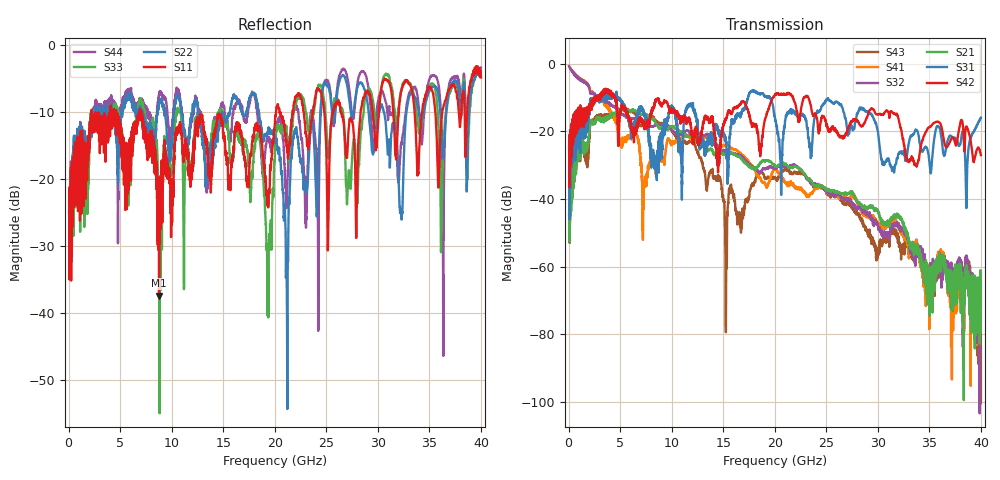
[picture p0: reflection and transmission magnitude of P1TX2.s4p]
!Agilent Technologies,N5245A,MY49151084,A.09.20.08
!Agilent N5245A: A.09.20.08
!Date: Thursday, March 01, 2012 10:31:57
!Correction: S11(Full 4 Port(1,2,3,4))
!S12(Full 4 Port(1,2,3,4))
!S13(Full 4 Port(1,2,3,4))
!S14(Full 4 Port(1,2,3,4))
!S21(Full 4 Port(1,2,3,4))
!S22(Full 4 Port(1,2,3,4))
!S23(Full 4 Port(1,2,3,4))
!S24(Full 4 Port(1,2,3,4))
!S31(Full 4 Port(1,2,3,4))
!S32(Full 4 Port(1,2,3,4))
!S33(Full 4 Port(1,2,3,4))
!S34(Full 4 Port(1,2,3,4))
!S41(Full 4 Port(1,2,3,4))
!S42(Full 4 Port(1,2,3,4))
!S43(Full 4 Port(1,2,3,4))
!S44(Full 4 Port(1,2,3,4))
!S4P File: Measurements: <S11,S12,S13,S14>,
!<S21,S22,S23,S24>,
!<S31,S32,S33,S34>,
!<S41,S42,S43,S44>:
# Hz S  dB  R 50
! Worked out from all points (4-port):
!   3996 points, 50 MHz to 40 GHz, reference 50 ohm
!   strongest paths, dB at 50 MHz, 10.04 GHz, 20.03 GHz, 30.02 GHz, 40 GHz:
!     S42: -25.3, -14.5, -9.1, -15.0, -27.0
!     S31: -25.3, -12.6, -16.3, -20.3, -15.9
!     S21: -44.5, -18.5, -30.1, -43.9, -71.4
!     S32: -0.8, -19.6, -30.9, -48.1, -68.8
!     S41: -0.7, -23.8, -31.1, -47.9, -64.7
!     S43: -44.8, -20.1, -33.5, -54.7, -100.3
!   lowest |S11| = -37.5 dB at 8.77 GHz (marker M1), VSWR 1.03, Z = 50.4 + j1.3 ohm
!   |S11| at or under -10 dB: start of sweep to 2.235 GHz; 4.581 GHz to 6.927 GHz (2.346 GHz wide, 40.8 % of centre); 7.031 GHz to 20.13 GHz (13.1 GHz wide, 96.5 % of centre)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
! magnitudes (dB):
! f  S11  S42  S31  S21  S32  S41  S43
! 50 MHz  -23.4  -25.3  -25.3  -44.5  -0.8  -0.7  -44.8
! 2.24 GHz  -9.7  -10.8  -10.6  -16.6  -8.8  -8.8  -16.7
! 8.77 GHz  -37.5  -11.0  -23.0  -19.0  -18.0  -28.3  -17.5
! 15.28 GHz  -16.4  -16.3  -23.7  -27.0  -25.6  -24.1  -59.5
! 21.15 GHz  -15.1  -9.2  -15.1  -29.9  -30.3  -35.3  -31.5
! 24.83 GHz  -10.4  -16.1  -11.7  -36.8  -37.3  -37.0  -37.2
! 40 GHz  -4.9  -27.0  -15.9  -71.4  -68.8  -64.7  -100.3
